TYPE APCControlAO :
STRUCT
	Zero_Reset_P1	:	REAL	;
	Zero_adjust_P1	:	REAL	;
	Span_adjust_P1	:	REAL	;
	Zero_Reset_P2	:	REAL	;
	Zero_adjust_P2	:	REAL	;
	Span_adjust_P2	:	REAL	;
	Slow_vacuum_control_target_vacuum_Pressure	:	REAL	;
	Valve_status_threshold	:	REAL	;
	Forbid_interlock_outbreak	:	REAL	;
	Slow_vacuum_mode_setting	:	REAL	;
	Interlock1	:	REAL	;
	Interlock2	:	REAL	;
	Interlock3	:	REAL	;
	Interlock_constant_of_interlock3	:	REAL	;
	P1_sensor_offset_setting	:	REAL	;
	Pos_mon_offset_setting	:	REAL	;
	Sensor_adjust_reset	:	REAL	;
	Slow_vacuum_rate	:	REAL	;
	Slow_vacuum_control_P	:	REAL	;
	Slow_vacuum_control_I	:	REAL	;
	Slow_vacuum_control_D	:	REAL	;
	Slow_vacuum_control_a	:	REAL	;
	controller_mode_select	:	REAL	;
	Specify_target_vacuum_Pressure_control	:	REAL	;
	Specify_target_opening_for_valve_opening_control	:	REAL	;
	Specify_control_mode	:	REAL	;
	Range_Upper_Limit_Sensor_Input1	:	REAL	;
	Range_Upper_Limit_Sensor_Input2	:	REAL	;

END_STRUCT
END_TYPE
